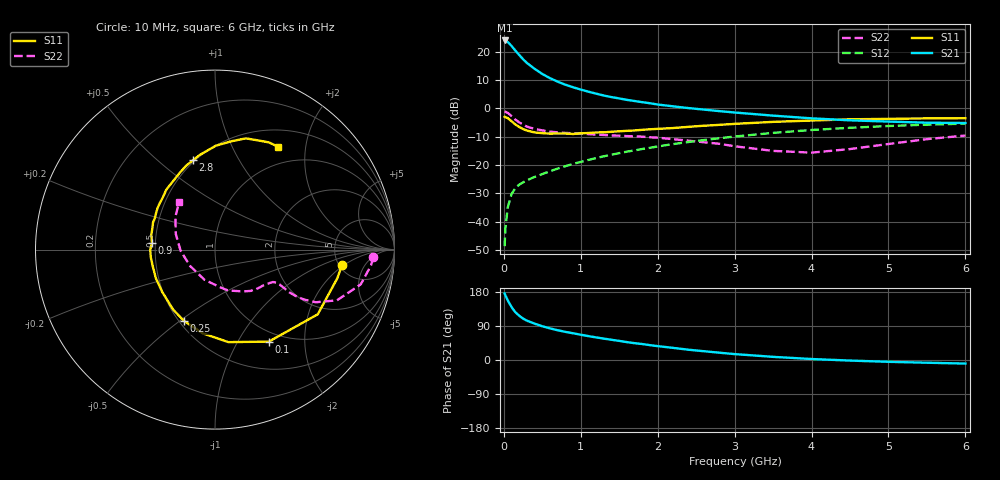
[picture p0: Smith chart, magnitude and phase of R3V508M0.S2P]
! SIEMENS Small Signal Semiconductors
! BFR181
! Si NPN RF Bipolar Junction Transistor in SOT23
! VCE = 0.5 V  IC = 8 mA
! Common Emitter S-Parameters:  May  1996
# GHz  S  MA  R  50
!  f  S11  S21  S12  S22
! GHz  MAG  ANG  MAG  ANG  MAG  ANG  MAG  ANG
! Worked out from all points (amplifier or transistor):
!   36 points, 10 MHz to 6 GHz, reference 50 ohm
!   highest |S21| = 24.0 dB at 10 MHz (marker M1)
!   |S21| within 3 dB of that: start of sweep to 132.4 MHz
!   unconditionally stable (mu >= 1): 309.2 MHz to end of sweep
!   at 250 MHz: K = 0.87, MSG = 21.7 dB, |S12| = -26.1 dB
!   at 1.4 GHz: K = 1.55, MAG = 5.8 dB, |S12| = -16.3 dB
!   at 6 GHz: K = 1.19, MAG = -2.5 dB, |S12| = -5.4 dB
!   S11 on the Smith chart (normalised r, x): 10 MHz: 5.33, -1.83; 100 MHz: 0.86, -1.36; 250 MHz: 0.53, -0.52; 900 MHz: 0.48, +0.04; 2.8 GHz: 0.49, +0.66; 6 GHz: 0.73, +1.53
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0.01  0.7133 -6.8  15.86 175.5  0.0037 85.5  0.883 -2.7
0.02  0.6999 -13.2  15.69 170.5  0.0075 83.0  0.8742 -5.7
0.05  0.6766 -32.2  14.92 157.7  0.0177 72.5  0.8349 -13.4
0.1  0.5939 -59.7  12.7 139.8  0.0308 63.3  0.7358 -22.6
0.15  0.5208 -81.8  10.5 126.0  0.0393 56.3  0.6332 -27.6
0.2  0.471 -98.6  8.788 116.8  0.0451 53.5  0.5679 -29.3
0.25  0.433 -113.6  7.386 109.3  0.0496 52.0  0.5163 -29.9
0.3  0.4075 -124.9  6.359 103.8  0.0538 52.2  0.4776 -29.9
0.4  0.377 -141.3  5.003 95.9  0.0618 53.2  0.4353 -29.0
0.5  0.366 -154.3  4.056 89.0  0.0694 55.0  0.4093 -28.4
0.6  0.3591 -164.7  3.425 83.5  0.0779 56.5  0.3903 -28.4
0.7  0.3607 -173.6  2.973 78.5  0.0866 57.7  0.3776 -28.8
0.9  0.3536 173.7  2.364 70.5  0.1046 59.2  0.3645 -30.0
1.1  0.3681 161.7  1.976 63.0  0.1232 60.0  0.3523 -32.4
1.3  0.3781 152.6  1.69 56.4  0.1429 59.8  0.3397 -35.2
1.6  0.4022 140.0  1.416 47.2  0.173 58.9  0.3248 -40.6
2.2  0.4507 120.2  1.089 32.0  0.2349 54.7  0.2865 -54.2
2.8  0.5129 103.8  0.897 19.3  0.2978 48.8  0.2378 -72.6
3.5  0.5791 89.5  0.746 8.3  0.3702 40.1  0.178 -109.2
4.5  0.6432 74.5  0.617 -1.5  0.4554 26.3  0.1918 -178.0
5.5  0.6683 63.4  0.56 -7.2  0.5171 12.8  0.287 140.2
6  0.6725 58.5  0.553 -9.4  0.5387 6.2  0.3322 127.0
